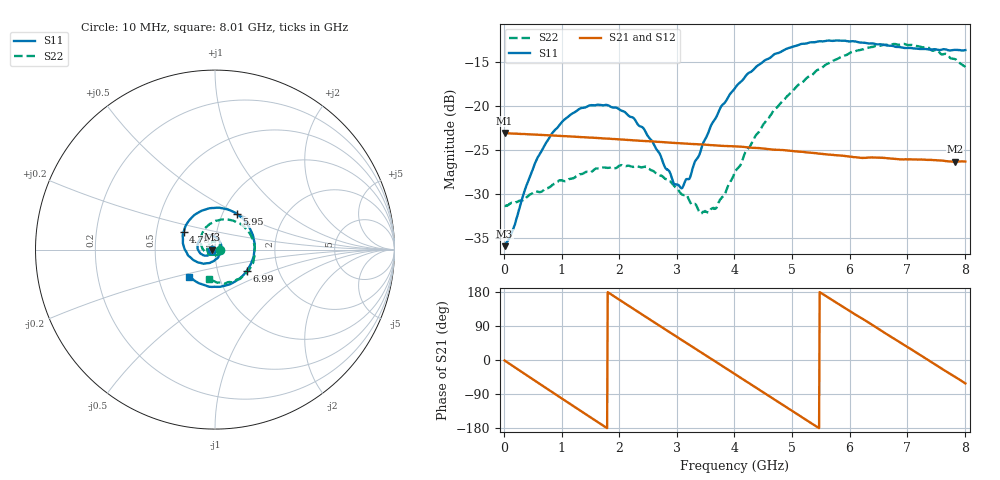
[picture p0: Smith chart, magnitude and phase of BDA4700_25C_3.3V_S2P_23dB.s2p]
!Agilent Technologies,E5071B,MY42404982,A.09.10
!Date: Mon Oct 20 18:12:43 2025
!Data & Calibration Information:
!Freq	S11:SOLT2(ON)	S21:SOLT2(ON)	S12:SOLT2(ON)	S22:SOLT2(ON)
# Hz S RI R 50
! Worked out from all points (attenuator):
!   801 points, 10 MHz to 8.01 GHz, reference 50 ohm
!   highest |S21| = -23.07 dB at 10 MHz (marker M1); lowest = -26.3 dB at 7.83 GHz (marker M2)
!   lowest |S11| = -35.9 dB at 10 MHz (marker M3), VSWR 1.03, Z = 48.4 - j0.106 ohm
!   |S11| at or under -10 dB: start of sweep to end of sweep
!   |S22| runs from -32.2 to -13.0 dB; largest |S21 - S12| = 0.00079
!   S11 on the Smith chart (normalised r, x): 10 MHz: 0.97, -0.00; 4.78 GHz: 0.69, +0.14; 5.95 GHz: 1.16, +0.49; 6.99 GHz: 1.38, -0.34; 8.01 GHz: 0.72, -0.23
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1e7  -0.016 -0.00109  0.0702 -0.00152  0.0702 -0.00159  0.0271 -0.000811
1.5e8  -0.0171 -0.00978  0.0671 -0.0187  0.0671 -0.0187  0.0272 -0.00736
6e8  -0.0402 -0.0329  0.0331 -0.06  0.0331 -0.06  0.0131 -0.0297
1.01e9  -0.0777 -0.0244  -0.0143 -0.0659  -0.0143 -0.0659  -0.0156 -0.0345
1.35e9  -0.0971 0.00649  -0.048 -0.0461  -0.048 -0.0461  -0.0369 -0.0179
2.08e9  -0.0505 0.078  -0.0565 0.0308  -0.0565 0.0308  -0.0298 0.0346
2.42e9  -0.00434 0.0746  -0.0296 0.0559  -0.0296 0.0559  -0.00418 0.0448
2.68e9  0.0239 0.0493  -0.0026 0.0624  -0.0027 0.0624  0.014 0.0381
2.95e9  0.0346 0.0105  0.0251 0.0562  0.0249 0.0562  0.0266 0.0231
3.09e9  0.0322 -0.0112  0.0376 0.0485  0.0371 0.0486  0.0291 0.0118
3.23e9  0.0233 -0.0316  0.0474 0.0382  0.0475 0.0381  0.0285 0.00163
3.54e9  -0.0159 -0.0677  0.0595 0.00894  0.0595 0.00882  0.0139 -0.0208
3.69e9  -0.0435 -0.0754  0.0593 -0.00625  0.0593 -0.00645  0.000975 -0.0265
4.01e9  -0.108 -0.0649  0.0469 -0.0358  0.0469 -0.0356  -0.0322 -0.0267
4.78e9  -0.1746 0.0986  -0.0218 -0.0519  -0.0214 -0.052  -0.0793 0.0635
5.35e9  -0.0665 0.2193  -0.053 -0.0109  -0.053 -0.0113  -0.0158 0.1488
5.95e9  0.1199 0.1997  -0.036 0.0374  -0.0361 0.0371  0.1207 0.1524
6.68e9  0.2186 -0.0181  0.0215 0.0456  0.0215 0.0456  0.2212 -0.00151
6.99e9  0.1765 -0.1184  0.0404 0.0291  0.0405 0.0289  0.205 -0.0853
7.45e9  0.0404 -0.2052  0.0488 -0.00722  0.0487 -0.00733  0.1111 -0.1727
7.83e9  -0.0912 -0.1867  0.0345 -0.0337  0.0345 -0.0338  0.0107 -0.1836
8.01e9  -0.1425 -0.1502  0.0228 -0.0426  0.023 -0.0426  -0.033 -0.1627
